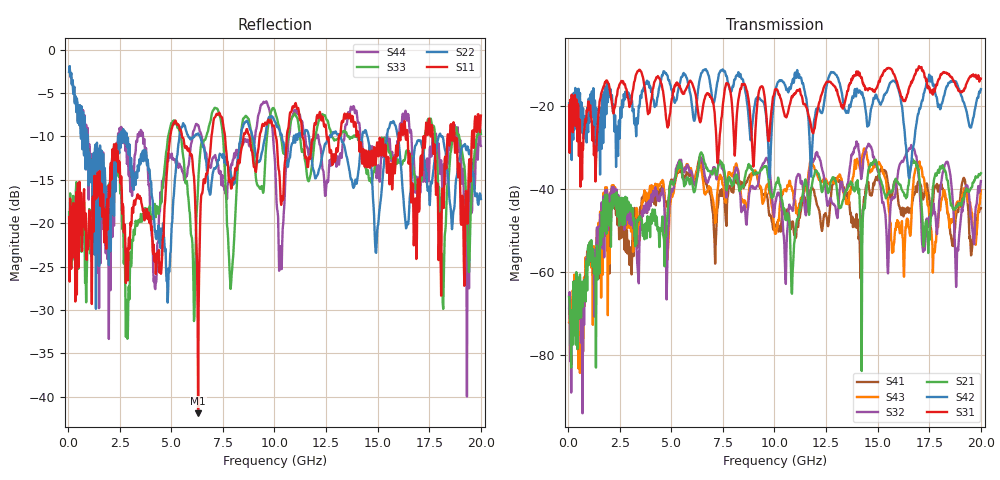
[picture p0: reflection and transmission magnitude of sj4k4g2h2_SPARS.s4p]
! FILE: E:\users\goganessyan\GBX_Backplane\FR408_backplane\1m_INBOUND_NEXT\sj4k4g2h2_SPARS.s4p
# MHZ S RI R 50.00
! FREQ  S11  S12  S13  S14
!  S21  S22  S23  S24
!  S31  S32  S33  S34
!  S41  S42  S43  S44
!  REAL  IMAG  REAL  IMAG  REAL  IMAG  REAL  IMAG
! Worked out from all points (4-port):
!   799 points, 50 MHz to 20 GHz, reference 50 ohm
!   strongest paths, dB at 50 MHz, 5.025 GHz, 10.03 GHz, 15.03 GHz, 20 GHz:
!     S31: -19.8, -18.2, -16.0, -14.7, -13.4
!     S42: -19.3, -16.0, -16.9, -18.4, -15.9
!     S21: -66.1, -38.1, -39.7, -35.2, -36.2
!     S32: -68.7, -40.1, -43.9, -35.9, -38.1
!     S43: -72.1, -41.7, -50.8, -33.6, -40.3
!     S41: -65.8, -37.7, -48.9, -36.7, -44.6
!   lowest |S11| = -41.9 dB at 6.3 GHz (marker M1), VSWR 1.02, Z = 49.8 - j0.775 ohm
!   |S11| at or under -10 dB: start of sweep to 4.945 GHz; 5.52 GHz to 6.947 GHz (1.427 GHz wide, 22.9 % of centre); 14.08 GHz to 16.01 GHz (1.932 GHz wide, 12.8 % of centre)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
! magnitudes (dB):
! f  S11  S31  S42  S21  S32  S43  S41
! 50 MHz  -19.3  -19.8  -19.3  -66.1  -68.7  -72.1  -65.8
! 6.3 GHz  -41.9  -21.4  -16.0  -35.4  -36.0  -34.6  -33.8
! 10.85 GHz  -6.9  -17.6  -14.5  -65.3  -44.6  -40.1  -48.7
! 12.03 GHz  -8.2  -22.7  -20.6  -35.7  -31.2  -35.7  -43.0
! 18.38 GHz  -10.2  -12.2  -15.2  -37.9  -33.4  -45.4  -45.8
! 18.82 GHz  -10.2  -15.4  -14.4  -44.3  -60.4  -43.4  -45.7
! 20 GHz  -7.6  -13.4  -15.9  -36.2  -38.1  -40.3  -44.6
